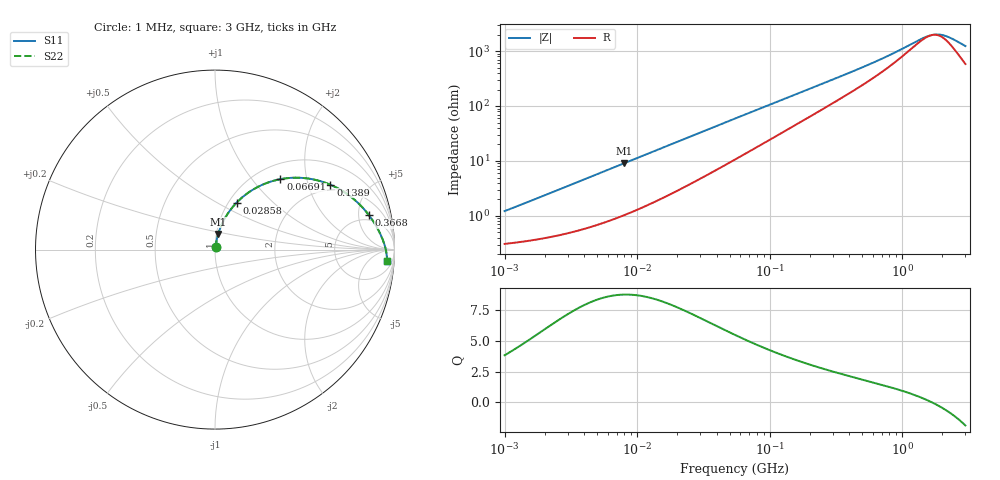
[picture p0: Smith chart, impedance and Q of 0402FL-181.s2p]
# MHz S MA R 50
!Freq  MagS11  AngS11  MagS21  AngS21  MagS12  AngS12  MagS22  AngS22
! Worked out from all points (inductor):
!   801 points, 1 MHz to 3 GHz, reference 50 ohm
!   read as one part in series: L = 187 nH near 1.041 MHz
!   highest Q = 8.76 at 7.938 MHz (marker M1), where L = 180 nH
!   self-resonance near 1.68 GHz
!   S11 on the Smith chart (normalised r, x): 1 MHz: 1.01, +0.02; 28.58 MHz: 1.09, +0.62; 66.91 MHz: 1.28, +1.41; 138.9 MHz: 1.76, +2.80; 366.8 MHz: 4.02, +6.77; 3 GHz: 13, -22
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1  0.01219 74.7  0.9968 -0.7  0.9968 -0.7  0.01219 74.7
3.823119  0.04405 80.2  0.9935 -2.5  0.9935 -2.5  0.04405 80.2
7.937891  0.0891 78.4  0.986 -5.1  0.986 -5.1  0.0891 78.4
14.47069  0.1572 74.2  0.9689 -9.0  0.9689 -9.0  0.1572 74.2
20.74721  0.2185 70.0  0.948 -12.5  0.948 -12.5  0.2185 70.0
28.57884  0.2887 65.2  0.9173 -16.6  0.9173 -16.6  0.2887 65.2
39.36673  0.3738 59.2  0.8702 -21.7  0.8702 -21.7  0.3738 59.2
54.77226  0.4733 51.9  0.8001 -27.7  0.8001 -27.7  0.4733 51.9
66.90963  0.5359 47.1  0.7466 -31.7  0.7466 -31.7  0.5359 47.1
94.97575  0.641 38.4  0.6371 -38.7  0.6371 -38.7  0.641 38.4
138.9236  0.7374 29.4  0.5085 -45.3  0.5085 -45.3  0.7374 29.4
209.4008  0.8139 21.0  0.3785 -50.6  0.3785 -50.6  0.8139 21.0
274.3666  0.8502 16.5  0.3046 -52.6  0.3046 -52.6  0.8502 16.5
366.7557  0.8795 12.5  0.2374 -53.4  0.2374 -53.4  0.8795 12.5
552.8145  0.909 8.1  0.1621 -51.9  0.1621 -51.9  0.909 8.1
792.5923  0.9272 5.0  0.1115 -46.8  0.1115 -46.8  0.9272 5.0
1430.499  0.9475 1.0  0.05524 -17.7  0.05524 -17.7  0.9475 1.0
1596.974  0.9503 0.3  0.04997 -6.1  0.04997 -6.1  0.9503 0.3
1747.494  0.9524 -0.2  0.04776 5.0  0.04776 5.0  0.9524 -0.2
1931.433  0.9545 -0.9  0.0479 18.0  0.0479 18.0  0.9545 -0.9
2156.205  0.9566 -1.6  0.0513 31.5  0.0513 31.5  0.9566 -1.6
3000  0.961 -3.9  0.07773 58.0  0.07773 58.0  0.961 -3.9
